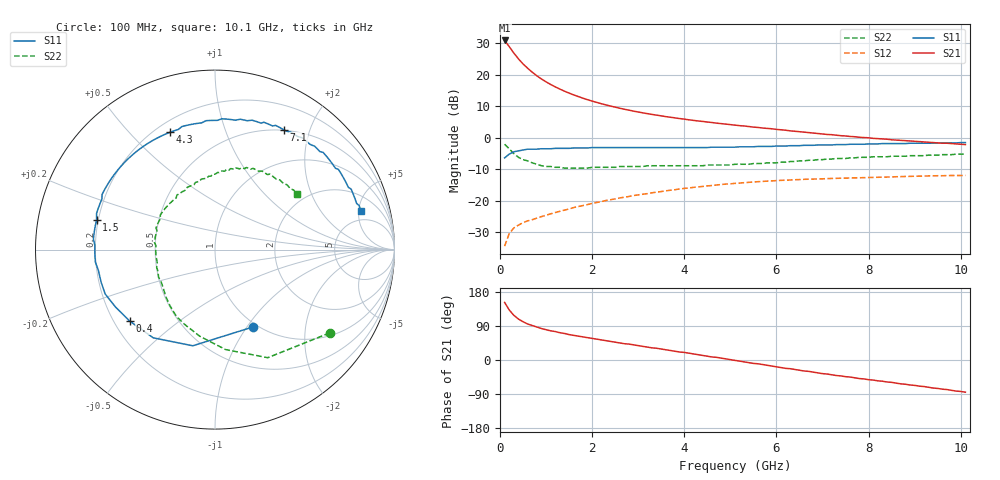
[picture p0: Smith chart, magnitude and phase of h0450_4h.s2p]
!HBFP-0450
!S and NOISE PARAMETERS at Vce=4V  Ic=50mA.  LAST UPDATED  09-04-98
# GHZ S MA R  50
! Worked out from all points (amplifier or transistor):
!   101 points, 100 MHz to 10.1 GHz, reference 50 ohm
!   highest |S21| = 30.9 dB at 100 MHz (marker M1)
!   |S21| within 3 dB of that: start of sweep to 251.1 MHz
!   unconditionally stable (mu >= 1): 2.248 GHz to end of sweep
!   at 1.7 GHz: K = 0.93, MSG = 17.5 dB, |S12| = -21.8 dB
!   at 5.1 GHz: K = 1.10, MAG = 7.4 dB, |S12| = -14.5 dB
!   at 10.1 GHz: K = 1.05, MAG = 3.5 dB, |S12| = -12.0 dB
!   lowest NFmin = 1.77 dB at 1.8 GHz
!   S11 on the Smith chart (normalised r, x): 100 MHz: 0.95, -1.07; 400 MHz: 0.26, -0.34; 1.5 GHz: 0.19, +0.12; 4.3 GHz: 0.26, +0.66; 7.1 GHz: 0.49, +1.62; 10.1 GHz: 3.55, +5.25
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0.1  0.48 -64.0  35.18 152.0  0.019 59.0  0.79 -36.0
0.2  0.55 -103.0  28.09 132.0  0.03 49.0  0.67 -64.0
0.3  0.6 -125.0  22.2 118.0  0.037 43.0  0.56 -84.0
0.4  0.62 -140.0  17.95 108.0  0.041 40.0  0.49 -100.0
0.5  0.64 -150.0  14.9 101.0  0.045 39.0  0.45 -112.0
0.6  0.66 -158.0  12.74 95.0  0.048 38.0  0.43 -120.0
0.7  0.66 -164.0  11.01 91.0  0.05 38.0  0.4 -129.0
0.8  0.66 -170.0  9.66 87.0  0.053 38.0  0.38 -136.0
0.9  0.67 -174.0  8.6 83.0  0.056 39.0  0.36 -143.0
1.1  0.67 178.0  7.03 77.0  0.062 40.0  0.35 -154.0
1.3  0.68 172.0  5.94 72.0  0.068 40.0  0.34 -163.0
1.5  0.68 166.0  5.13 67.0  0.074 40.0  0.33 -171.0
1.8  0.69 158.0  4.26 61.0  0.084 39.0  0.33 179.0
2.2  0.7 150.0  3.48 53.0  0.097 37.0  0.34 168.0
2.6  0.7 142.0  2.95 45.0  0.111 33.0  0.35 160.0
3.5  0.7 125.0  2.23 29.0  0.14 25.0  0.36 143.0
4.3  0.7 111.0  1.85 14.0  0.166 15.0  0.36 129.0
5.1  0.71 96.0  1.59 -1.0  0.189 4.0  0.38 114.0
6.8  0.76 65.0  1.19 -32.0  0.221 -21.0  0.44 83.0
7.1  0.77 60.0  1.13 -37.0  0.225 -25.0  0.46 79.0
8.5  0.81 39.0  0.93 -59.0  0.239 -44.0  0.51 59.0
10.1  0.84 15.0  0.78 -85.0  0.252 -67.0  0.55 34.0
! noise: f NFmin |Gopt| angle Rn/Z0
1.8  1.77  0.6  -151  0.1
2  1.81  0.6  -149  0.11
2.5  1.94  0.61  -139  0.17
3.5  2.23  0.63  -123  0.34
4  2.37  0.66  -112  0.49
4.5  2.51  0.68  -104  0.65
5.5  2.79  0.71  -84  1.19
6  2.93  0.72  -75  1.48
7  3.21  0.76  -57  2.39
9  3.78  0.81  -26  4.3
